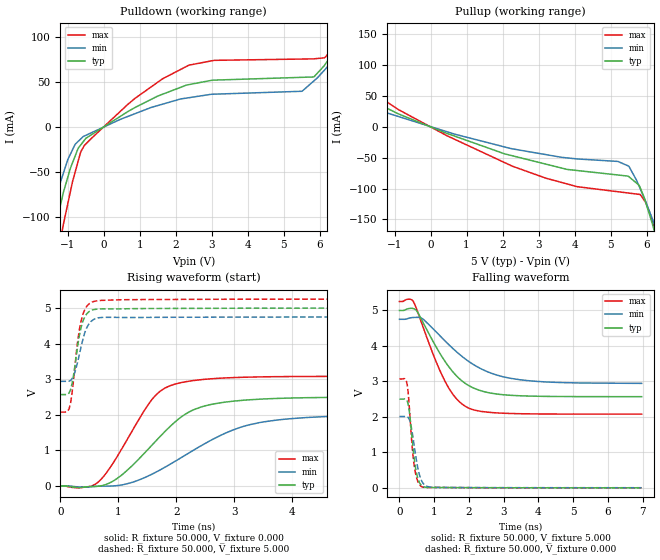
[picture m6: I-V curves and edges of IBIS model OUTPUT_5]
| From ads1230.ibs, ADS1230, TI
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|   Output OUTPUT 5V Model
[Model]   OUTPUT_5
Model_type Output
|Signal _DRDY_DOUT(16) pin
Polarity   Non-Inverting
Enable   Active-Low
Vmeas = 2.5
Vref = 2.5
Cref = 15pF
Rref = 50
|   typ   min   max
|   (nom PVT)   (Fast PVT)   (slow PVT)
|Average
C_comp   3.684e-12   3.413e-12   4.817e-12
|ON state : BUFFER OUTPUT TURNED HIGH
|C_comp   4.263e-12   3.767e-12   5.422e-12
|OFF state: BUFFER in HIGH IMPEDANCE for IOs and 3-state,
|This is BUFFER in LOW state for OUTPUT only type
|C_comp   3.104e-12   3.060e-12   4.212e-12
| Where   nom PVT is  Nominal Process, 5.0V, 25C
|   Fast PVT is Strong Process, 5.25V, -40C
|   Slow PVT is Weak Process, 4.75V, 85C
[Voltage Range]   5   4.75   5.25
|Ambient Temperature   25   85   -40
|Junction Temperature
[Temperature Range]   25   85   -40
[Pullup Reference]   5   4.75   5.25
[Pulldown Reference]   0   0   0
[Power Clamp Reference]   5   4.75   5.25
[GND Clamp Reference]   0   0   0
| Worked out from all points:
|   slope of the pulldown table from 0 to 0.75 V, typ, clamps not added: 39.7 ohm
|   slope of the pullup table from 0 to 0.75 V, typ, clamps not added: 45 ohm
|   falling waveform, R_fixture 50.000, V_fixture 5.000: 20-80 % time 993ps typ, 1.4ns min, 835ps max; typ from 5 V to 2.57 V
|   rising waveform, R_fixture 50.000, V_fixture 0.000: 20-80 % time 949ps typ, 1.37ns min, 701ps max; typ from 0.001 V to 2.5 V
|   rising waveform, R_fixture 50.000, V_fixture 5.000: 20-80 % time 146ps typ, 171ps min, 146ps max; typ from 2.57 V to 5 V
|   falling waveform, R_fixture 50.000, V_fixture 0.000: 20-80 % time 171ps typ, 205ps min, 157ps max; typ from 2.5 V to 0.001 V
[Pulldown]
|   Voltage   I(typ)   I(min)   I(max)
-5V       -968.8mA   -712.8mA   -1.388A
-1.625V   -175.3mA   -125.1mA   -254.6mA
-1.33V    -112.5mA   -80.54mA   -162.4mA
-1.141V   -76.87mA   -54.23mA   -113.2mA
-801mV    -33.31mA   -20.05mA   -51.59mA
-537.5mV  -14.89mA   -10.14mA   -20.71mA
880mV     21.81mA    14.89mA    32.04mA
2.371V    47.11mA    32.54mA    68.78mA
5.507V    55.2mA     39.68mA    75.54mA
6.13V     68.33mA    63.11mA    76.93mA
7.217V    131.3mA    112.1mA    156.3mA
10V       253.9mA    206.6mA    324.7mA
[Pullup]
|   Voltage   I(typ)   I(min)   I(max)
-5V       246.8mA    196.9mA    326.5mA
-4.879V   203.2mA    165.4mA    258.1mA
-4.569V   162.8mA    135.4mA    202.7mA
-3.525V   127.2mA    104.8mA    162.1mA
-1.224V   30.72mA    22.98mA    41.01mA
2.282V    -46.89mA   -35.63mA   -63.87mA
4.077V    -70.73mA   -51.93mA   -96.96mA
5.502V    -80.38mA   -63.48mA   -107.3mA
5.825V    -98.98mA   -100.5mA   -109.6mA
6.16V     -156.9mA   -148.9mA   -151.9mA
6.282V    -182.6mA   -167.5mA   -178mA
10V       -1.056A    -820.1mA   -1.417A
[Ramp]
R_load = 50
|   typ   min   max
dV/dt_r   1.52721/9.47379e-10   1.22391/1.37107e-09   1.85013/7.00622e-10
dV/dt_f   1.47588/9.92584e-10   1.08384/1.39478e-09   1.90331/8.35729e-10
[Falling Waveform]
R_fixture = 50.000
V_fixture = 5.000
V_fixture_min = 4.750
V_fixture_max = 5.250
C_fixture = 0.000
|  time   V(typ)   V(min)   V(max)
0s        4.998V     4.75V      5.25V
400ps     5.052V     4.801V     5.25V
675ps     4.67V      4.758V     4.546V
1.025ns   4.026V     4.427V     3.631V
1.325ns   3.546V     4.13V      2.981V
1.625ns   3.175V     3.851V     2.531V
2ns       2.88V      3.559V     2.245V
2.675ns   2.663V     3.22V      2.121V
3.45ns    2.596V     3.049V     2.09V
6.975ns   2.569V     2.944V     2.078V
[Rising Waveform]
R_fixture = 50.000
V_fixture = 0.000
V_fixture_min = 0.000
V_fixture_max = 0.000
C_fixture = 0.000
|  time   V(typ)   V(min)   V(max)
0s        1.184mV    4.249mV    1.215nV
325ps     -41.81mV   -26.38mV   -49.41mV
650ps     -5.09mV    -6.568mV   109.8mV
1.05ns    299.2mV    29mV       1.021V
1.575ns   1.14V      329.6mV    2.422V
1.975ns   1.795V     690.2mV    2.861V
2.5ns     2.253V     1.198V     2.999V
2.975ns   2.382V     1.572V     3.045V
3.5ns     2.445V     1.8V       3.067V
6.975ns   2.502V     2.011V     3.084V
[Rising Waveform]
R_fixture = 50.000
V_fixture = 5.000
V_fixture_min = 4.750
V_fixture_max = 5.250
C_fixture = 0.000
|  time   V(typ)   V(min)   V(max)
0s        2.569V     2.941V     2.077V
150ps     2.617V     2.946V     2.172V
200ps     2.873V     3.012V     2.606V
250ps     3.376V     3.202V     3.358V
300ps     3.963V     3.506V     4.101V
350ps     4.415V     3.867V     4.595V
400ps     4.683V     4.199V     4.881V
450ps     4.829V     4.433V     5.04V
575ps     4.955V     4.68V      5.184V
6.975ns   4.998V     4.75V      5.25V
[Falling Waveform]
R_fixture = 50.000
V_fixture = 0.000
V_fixture_min = 0.000
V_fixture_max = 0.000
C_fixture = 0.000
|  time   V(typ)   V(min)   V(max)
0s        2.502V     2.011V     3.069V
150ps     2.506V     2.011V     3.077V
225ps     2.443V     2.003V     2.902V
275ps     2.234V     1.949V     2.407V
325ps     1.803V     1.799V     1.705V
425ps     834.8mV    1.19V      632.3mV
525ps     283.9mV    584.7mV    192.9mV
650ps     56.09mV    175.7mV    29.71mV
1.025ns   10.79mV    14.4mV     12.24mV
6.975ns   1.184mV    4.249mV    268.5uV
